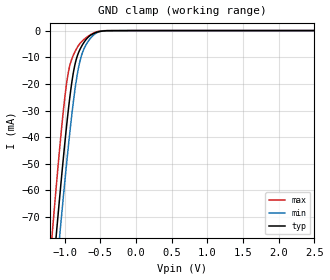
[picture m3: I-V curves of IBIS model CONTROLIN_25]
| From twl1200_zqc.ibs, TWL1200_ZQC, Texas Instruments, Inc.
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[Model]   CONTROLIN_25
Model_type  Input
Vinl=0.875
Vinh=1.625
| variable   typ   min   max
C_comp   1.84pF   1.49pF   2.48pF
[Temperature Range]   40   100   -40
| Ambient temperature   25   85   -40
[Voltage range]   2.5   2.3   2.7
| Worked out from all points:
|   GND clamp passes 1 mA (typ) near -0.59 V on its own axis
[GND Clamp]
| CONTROLIN_25
|   Voltage   I(typ)   I(min)   I(max)
-2.5V     -537.5mA   -541.2mA   -533.3mA
-1.175V   -94.8mA    -108.9mA   -76.9mA
-1.115V   -76.42mA   -90.86mA   -58.14mA
-1.065V   -61.57mA   -76.14mA   -43.25mA
-1.01V    -45.98mA   -60.47mA   -28.38mA
-960mV    -32.92mA   -46.91mA   -17.75mA
-865mV    -14.13mA   -24.32mA   -8.532mA
-810mV    -8.688mA   -14.72mA   -5.81mA
-760mV    -5.839mA   -9.142mA   -4.117mA
-615mV    -1.388mA   -2.223mA   -1.219mA
-405mV    -39.34uA   -49.73uA   -10.06uA
2.5V      156.4pA    883.8pA    34.32pA
